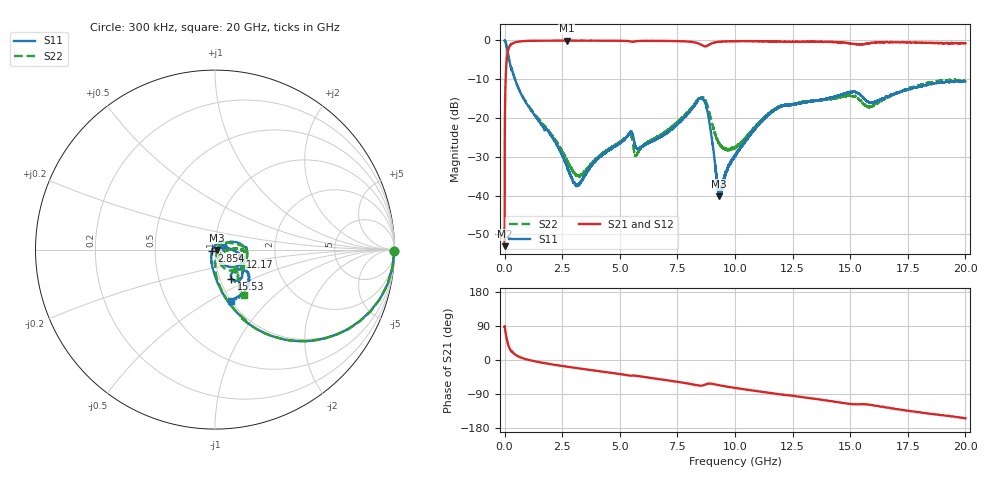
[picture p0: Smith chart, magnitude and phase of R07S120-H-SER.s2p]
!{R07S120}
!Johanson Technology Inc.
!www.johansontechnology.com
!Test Board Conditions:
!Substrate Type  RO4350B
!Substrate Thickness  10 mil
!Substrate Dk  3.66
!TL Type: GCPW
!TL Trace Width  21 mil
!TL Gap  20 mil
!Electrode orientation  Horizontal
!DUT TOPOLOGY	SERIES
!Mounting Pad LxW  16x21 mil
! Created Sat Feb  6 11:44:47 2021
# hz S ma R 50
! 2 Port Network Data from SP1.SP block
! freq  magS11  angS11  magS21  angS21  magS12  angS12  magS22  angS22
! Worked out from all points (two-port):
!   20001 points, 300 kHz to 20 GHz, reference 50 ohm
!   highest |S21| = -0.03 dB at 2.694 GHz (marker M1); lowest = -53.0 dB at 300 kHz (marker M2)
!   |S21| within 3 dB of the highest: 135 MHz to end of sweep
!   lowest |S11| = -40.2 dB at 9.307 GHz (marker M3), VSWR 1.02, Z = 50.9 - j0.276 ohm
!   |S11| at or under -10 dB: 448.2 MHz to end of sweep
!   |S22| runs from -35.1 to 0.0 dB; largest |S21 - S12| = 0.014
!   S11 on the Smith chart (normalised r, x): 300 kHz: open; 2.854 GHz: 0.97, -0.01; 12.17 GHz: 1.32, -0.10; 15.53 GHz: 1.13, -0.39; 20 GHz: 1.00, -0.63
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300000  1 -0.4  0.00223 88.2  0.002306 87.4  0.9986 -0.4
1.053e8  0.786 -39.0  0.6142 51.3  0.6152 51.2  0.7869 -38.9
2.283e8  0.5097 -61.6  0.8577 28.7  0.8567 28.8  0.5089 -61.6
7.533e8  0.1949 -84.6  0.9784 5.5  0.9781 5.5  0.1972 -83.3
2.6943e9  0.0243 -140.2  0.9962 -17.5  0.9947 -17.5  0.02905 -70.4
2.8543e9  0.01814 -156.1  0.9945 -18.9  0.9951 -18.9  0.0232 -58.6
3.0793e9  0.01387 168.3  0.9947 -20.9  0.9953 -20.8  0.01862 -34.1
3.3343e9  0.01533 125.0  0.9945 -23.1  0.9944 -23.0  0.01872 -2.0
5.4383e9  0.06488 21.8  0.9741 -41.2  0.9737 -41.1  0.06116 44.5
5.7153e9  0.04137 5.3  0.9781 -41.7  0.9785 -41.6  0.03284 49.8
6.6673e9  0.0554 26.3  0.9875 -50.2  0.9871 -50.2  0.05783 45.6
8.5933e9  0.1777 -16.8  0.8606 -67.4  0.8608 -67.4  0.1843 -20.0
8.8613e9  0.09914 -59.2  0.8754 -62.3  0.8766 -62.3  0.1252 -60.7
9.3073e9  0.00975 -16.1  0.9619 -66.5  0.9622 -66.6  0.04787 -62.7
1.00003e10  0.0326 34.8  0.979 -73.6  0.9782 -73.7  0.0423 -28.4
1.11623e10  0.09178 0.5  0.9762 -83.9  0.9769 -84.0  0.09512 1.6
1.21673e10  0.1462 -15.3  0.96 -92.2  0.9588 -92.1  0.1476 -1.2
1.33343e10  0.1642 -24.4  0.963 -101.3  0.9639 -101.5  0.1654 -3.4
1.49713e10  0.2163 -46.9  0.92 -115.6  0.9198 -115.7  0.1948 -30.5
1.55323e10  0.1881 -61.2  0.8949 -116.8  0.8913 -116.7  0.1575 -49.2
1.66673e10  0.1883 -34.3  0.9435 -125.9  0.9474 -126.3  0.1886 -47.6
2e10  0.2985 -72.8  0.9215 -153.7  0.9202 -153.6  0.3011 -57.6
